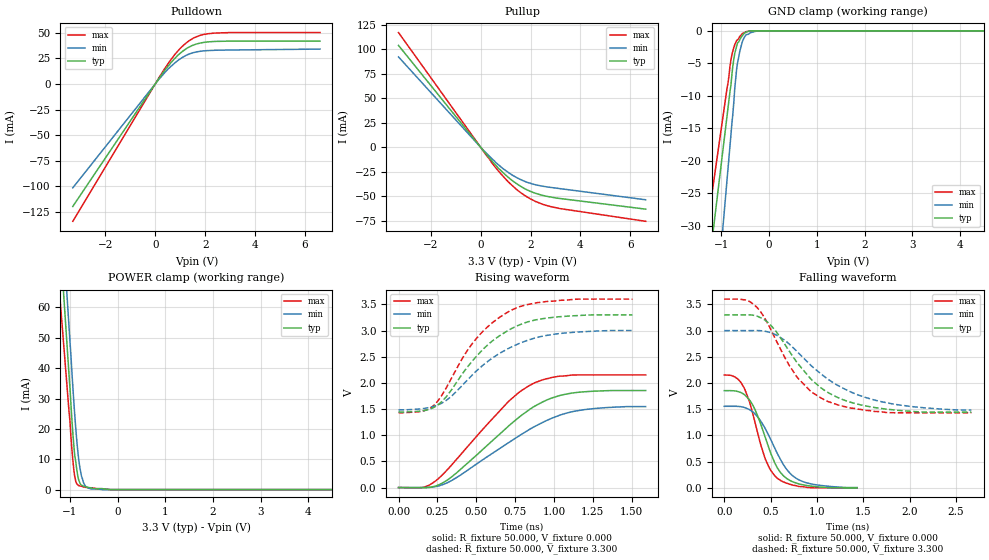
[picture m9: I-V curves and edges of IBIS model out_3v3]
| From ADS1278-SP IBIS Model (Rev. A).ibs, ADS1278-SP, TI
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[Model]   out_3v3
Model_type Output
Vref=0.000E+00
Rref=1.000E+06
Cref=2.000E-11
Vmeas=1.650E+00
C_comp   853.00E-15   853.00E-15   853.00E-15
[Voltage Range]   3.300E+00   3.000E+00   3.600E+00
[POWER Clamp Reference]   3.300E+00   3.000E+00   3.600E+00
[GND Clamp Reference]   0.000E+00   0.000E+00   0.000E+00
[Pullup Reference]   3.300E+00   3.000E+00   3.600E+00
[Pulldown Reference]   0.000E+00   0.000E+00   0.000E+00
[Temperature Range]   25   105   -40
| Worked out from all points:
|   slope of the pulldown table from 0 to 0.495 V, typ, clamps not added: 29.6 ohm
|   slope of the pullup table from 0 to 0.495 V, typ, clamps not added: 32.4 ohm
|   GND clamp passes 1 mA (typ) near -0.58 V on its own axis
|   POWER clamp passes 1 mA (typ) near -0.68 V on its own axis
|   rising waveform, R_fixture 50.000, V_fixture 0.000: 20-80 % time 431ps typ, 489ps min, 396ps max; typ from 0 V to 1.85 V
|   falling waveform, R_fixture 50.000, V_fixture 0.000: 20-80 % time 243ps typ, 288ps min, 218ps max; typ from 1.85 V to 0 V
|   rising waveform, R_fixture 50.000, V_fixture 3.300: 20-80 % time 338ps typ, 379ps min, 312ps max; typ from 1.44 V to 3.3 V
|   falling waveform, R_fixture 50.000, V_fixture 3.300: 20-80 % time 543ps typ, 692ps min, 460ps max; typ from 3.3 V to 1.44 V
[GND Clamp]
-3.3V     -160.3mA   -228.1mA   -133.3mA
-880mV    -12.98mA   -22.75mA   -8.748mA
-800mV    -8.376mA   -15.99mA   -4.467mA
-780mV    -6.74mA    -14.24mA   -3.716mA
-740mV    -4.348mA   -11mA      -2.549mA
-720mV    -3.483mA   -8.866mA   -2.141mA
-680mV    -2.341mA   -5.828mA   -1.491mA
-620mV    -1.454mA   -3.337mA   -922.2uA
-560mV    -726.3uA   -1.634mA   -407.4uA
-480mV    -203.1uA   -594.6uA   -134.7uA
-240mV    0A         0A         0A
6.6V      0A         0A         0A
[Power Clamp]
-3.3V     575.7mA    610.2mA    474.6mA
-1.02V    37.73mA    53.57mA    25.68mA
-1V       33.45mA    48.69mA    22.36mA
-960mV    23.07mA    38.73mA    13.28mA
-920mV    14.61mA    29.05mA    6.545mA
-900mV    11.18mA    24.51mA    4.283mA
-880mV    9.261mA    20.34mA    2.802mA
-820mV    3.338mA    10.34mA    1.339mA
-760mV    1.474mA    4.459mA    1.105mA
-720mV    1.182mA    2.445mA    862.4uA
-560mV    542.6uA    230.4uA    616.3uA
6.62V     0A         0A         0A
[Pullup]
-3.3V     103.8mA    92.09mA    116.9mA
120mV     -3.813mA   -3.238mA   -4.313mA
440mV     -13.32mA   -11.26mA   -15.6mA
720mV     -21.46mA   -17.97mA   -24.38mA
1.12V     -30.82mA   -25.74mA   -35.48mA
1.52V     -38.38mA   -31.81mA   -44.53mA
1.84V     -43.04mA   -35.37mA   -50.16mA
2.2V      -46.78mA   -38.07mA   -55.14mA
2.88V     -50.9mA    -41.03mA   -60.77mA
6.62V     -62.91mA   -53.37mA   -75.29mA
[Pulldown]
-3.3V     -119.5mA   -101.3mA   -134mA
200mV     7.228mA    6.06mA     8.208mA
540mV     18.15mA    15.24mA    20.72mA
760mV     24.31mA    19.99mA    27.96mA
1.02V     30.41mA    24.86mA    35.21mA
1.32V     35.58mA    28.86mA    41.59mA
1.52V     37.94mA    30.56mA    44.67mA
1.8V      39.95mA    31.9mA     47.44mA
2.36V     41.52mA    32.88mA    49.67mA
6.6V      41.92mA    34.08mA    50.21mA
[Rising Waveform]
R_fixture = 50.000
V_fixture = 0.000
V_fixture_min = 0.000
V_fixture_max = 0.000
|  time   V(typ)   V(min)   V(max)
0s        0V         0V         0V
155ps     -2.1mV     -199.8uV   1.98mV
237.5ps   28.17mV    17.78mV    124.2mV
372.5ps   278mV      189.4mV    536.7mV
702.5ps   1.16V      847.2mV    1.629V
780ps     1.355V     996.4mV    1.829V
877.5ps   1.557V     1.169V     2.004V
985ps     1.71V      1.323V     2.103V
1.13ns    1.811V     1.457V     2.151V
1.59ns    1.854V     1.547V     2.152V
[Falling Waveform]
R_fixture = 50.000
V_fixture = 0.000
V_fixture_min = 0.000
V_fixture_max = 0.000
|  time   V(typ)   V(min)   V(max)
0s        1.854V     1.556V     2.152V
172.5ps   1.823V     1.55V      2.027V
225ps     1.767V     1.529V     1.869V
282.5ps   1.653V     1.482V     1.584V
362.5ps   1.366V     1.349V     1.036V
445ps     953.3mV    1.123V     542mV
572.5ps   383.2mV    658.5mV    184.4mV
677.5ps   174.3mV    344.4mV    87.39mV
820ps     69.65mV    141.5mV    24.91mV
1.435ns   0V         6.578mV    0V
[Rising Waveform]
R_fixture = 50.000
V_fixture = 3.300
V_fixture_min = 3.000
V_fixture_max = 3.600
|  time   V(typ)   V(min)   V(max)
0s        1.444V     1.485V     1.432V
160ps     1.469V     1.51V      1.464V
227.5ps   1.532V     1.552V     1.571V
342.5ps   1.873V     1.749V     2.099V
420ps     2.211V     1.983V     2.515V
497.5ps   2.496V     2.219V     2.836V
602.5ps   2.799V     2.471V     3.146V
730ps     3.042V     2.691V     3.395V
1.01ns    3.257V     2.933V     3.565V
1.505ns   3.3V       3V         3.6V
[Falling Waveform]
R_fixture = 50.000
V_fixture = 3.300
V_fixture_min = 3.000
V_fixture_max = 3.600
|  time   V(typ)   V(min)   V(max)
0s        3.3V       3V         3.6V
262.5ps   3.3V       3V         3.564V
452.5ps   3.183V     2.983V     3.19V
652.5ps   2.743V     2.817V     2.491V
795ps     2.369V     2.585V     2.092V
937.5ps   2.074V     2.334V     1.837V
1.12ns    1.819V     2.073V     1.647V
1.37ns    1.63V      1.826V     1.52V
1.693ns   1.515V     1.645V     1.452V
2.668ns   1.444V     1.485V     1.432V
[Ramp]
dV/dt_r   1.112E+00/4.306E-10   9.295E-01/4.881E-10   1.292E+00/3.947E-10
dV/dt_f   1.114E+00/5.431E-10   9.089E-01/6.933E-10   1.301E+00/4.601E-10
R_load = 50
